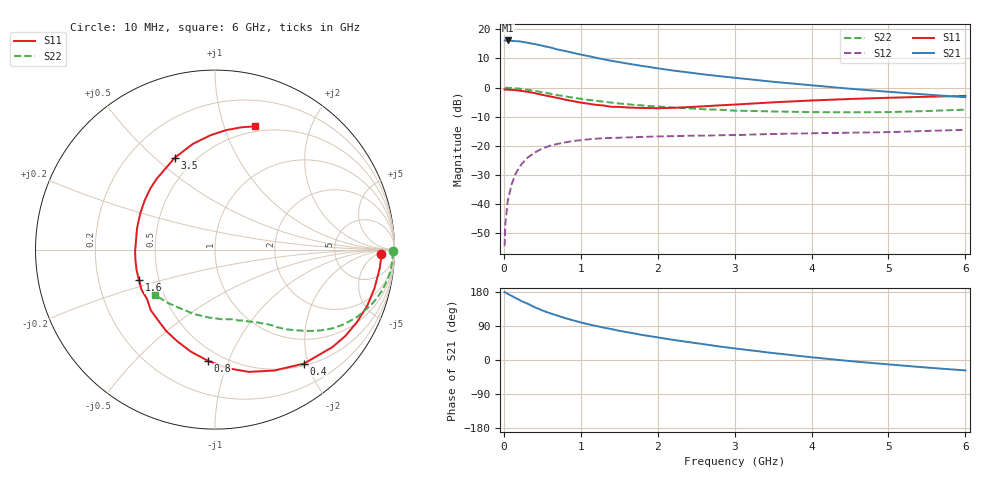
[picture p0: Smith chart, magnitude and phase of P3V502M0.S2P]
! SIEMENS Small Signal Semiconductors
! BFP181
! Si NPN RF Bipolar Junction Transistor in SOT143
! VCE = 0.5 V  IC = 2 mA
! Common Emitter S-Parameters:  March  1996
# GHz  S  MA  R  50
!  f  S11  S21  S12  S22
! GHz  MAG  ANG  MAG  ANG  MAG  ANG  MAG  ANG
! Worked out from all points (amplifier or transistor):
!   36 points, 10 MHz to 6 GHz, reference 50 ohm
!   highest |S21| = 16.2 dB at 50 MHz (marker M1)
!   |S21| within 3 dB of that: start of sweep to 685.8 MHz
!   unconditionally stable (mu >= 1): 2.016 GHz to end of sweep
!   at 250 MHz: K = 0.15, MSG = 20.7 dB, |S12| = -25.7 dB
!   at 1.4 GHz: K = 0.75, MSG = 13.2 dB, |S12| = -17.2 dB
!   at 6 GHz: K = 1.37, MAG = 2.0 dB, |S12| = -14.5 dB
!   S11 on the Smith chart (normalised r, x): 10 MHz: 22, -8; 400 MHz: 0.53, -1.93; 800 MHz: 0.42, -0.85; 1.6 GHz: 0.39, -0.17; 3.5 GHz: 0.39, +0.58; 6 GHz: 0.45, +1.27
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0.01  0.9239 -1.6  6.436 179.2  0.0019 89.2  0.992 -0.6
0.02  0.9263 -2.9  6.392 178.5  0.0046 85.3  0.9901 -1.4
0.05  0.9238 -6.5  6.445 174.7  0.0112 88.5  0.9898 -3.5
0.1  0.9142 -13.7  6.348 169.4  0.0216 80.9  0.9853 -7.0
0.2  0.8882 -27.1  6.233 158.7  0.043 72.9  0.9592 -13.6
0.25  0.8711 -33.6  6.068 153.6  0.052 69.5  0.9413 -16.8
0.4  0.8058 -52.0  5.607 139.4  0.0766 59.0  0.8776 -25.2
0.5  0.7504 -63.9  5.226 130.9  0.09 52.8  0.8336 -29.8
0.6  0.7069 -74.5  4.907 123.5  0.1004 47.7  0.7885 -33.8
0.7  0.6642 -84.1  4.508 116.8  0.1086 43.0  0.7439 -37.2
0.8  0.6206 -93.6  4.236 110.4  0.1149 39.2  0.7064 -39.9
1  0.5533 -112.1  3.68 99.2  0.1253 32.7  0.6417 -44.5
1.1  0.5293 -120.8  3.47 94.1  0.1294 30.0  0.6161 -46.5
1.3  0.4919 -136.7  3.055 85.4  0.1352 25.6  0.572 -49.9
1.6  0.4566 -158.1  2.595 73.5  0.14 21.1  0.5205 -53.8
1.8  0.4471 -172.4  2.35 66.1  0.1428 18.8  0.4948 -56.5
2.2  0.4502 164.8  1.963 53.2  0.1468 14.9  0.4548 -62.2
2.8  0.4955 136.7  1.573 35.7  0.1522 10.9  0.4171 -71.4
3.5  0.5585 113.7  1.259 18.3  0.1603 7.8  0.39 -84.5
4.5  0.638 92.2  0.957 -2.9  0.1684 2.6  0.3776 -107.7
5.5  0.6963 78.0  0.758 -20.0  0.1805 0.3  0.3966 -131.4
6  0.7215 72.1  0.684 -27.5  0.1888 -1.9  0.4186 -142.8
